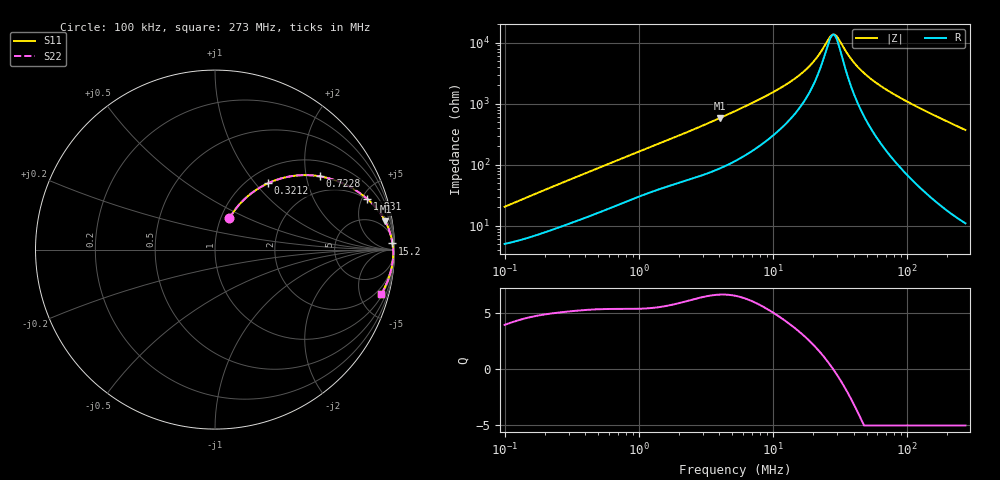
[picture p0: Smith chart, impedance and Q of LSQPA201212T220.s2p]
! LSQPA201212T220  S-PARAMETER MODEL  ( General Type )
! Model Generated by TAIYO YUDEN Corporation (http://www.ty-top.com)
! Version 2.0
! TAIYO YUDEN Control No. 100810NF17SB-FAC
! Copyright(c) 2007 TAIYO YUDEN CO.,LTD. All Rights Reserved.
! Product Description (link to TY-COMPAS)
! https://ds.yuden.co.jp/TYCOMPAS/or/detail?pn=LSQPA201212T220K&u=M
! Products Name : Inductors
! Characteristics :
!  Inductance : 22 uH , SRF(min) : 16 MHz , DC Resistance(max) : 4.81 Ohm
!  Rated Current : Saturation :170 mA , Temp Rise : 190 mA (40 degC)
!  Case Size : 2.0 x 1.25 / 0.079 x 0.049 [mm/inch] , Thickness : 1.25 / 0.049 [mm/inch]
!  (Conditions: Temperature = 25 degC , DC Bias Current/Voltage = 0A / 0V)
! External Node Assignments :
!  1  o---GGG---o  2
! GND o---------o GND
! Frequency Range : 0.1MHz  -  272.98108MHz  [ 402 STEP ]
# MHz S RI R 50
! Freq[MHz].  S11 Real  S11 Imag  S21 Real  S21 Imag  S12 Real  S12 Imag  S22 Real  S22 Imag
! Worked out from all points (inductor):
!   401 points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, 100 kHz to 273 MHz, reference 50 ohm
!   read as one part in series: L = 31.2 uH near 104 kHz
!   highest Q = 6.63 at 4.04 MHz (marker M1), where L = 22.8 uH
!   self-resonance near 28.07 MHz
!   S11 on the Smith chart (normalised r, x): 100 kHz: 1.10, +0.40; 321.2 kHz: 1.23, +1.17; 722.8 kHz: 1.45, +2.41; 1.831 MHz: 1.95, +5.48; 15.2 MHz: 16, +53; 273 MHz: 1.22, -7.41
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0.1  0.0807 0.1735  0.9193 -0.1735  0.9193 -0.1735  0.0807 0.1735
0.184629  0.1595 0.2765  0.8405 -0.2765  0.8405 -0.2765  0.1595 0.2765
0.32124  0.2956 0.3696  0.7044 -0.3696  0.7044 -0.3696  0.2956 0.3696
0.376316  0.3466 0.3899  0.6534 -0.3899  0.6534 -0.3899  0.3466 0.3899
0.722825  0.5858 0.408  0.4142 -0.408  0.4142 -0.408  0.5858 0.408
1.416134  0.7918 0.3253  0.2082 -0.3253  0.2082 -0.3253  0.7918 0.3253
1.831381  0.8478 0.2828  0.1522 -0.2828  0.1522 -0.2828  0.8478 0.2828
4.040099  0.9493 0.1566  0.0507 -0.1566  0.0507 -0.1566  0.9493 0.1566
5.329134  0.9654 0.1213  0.0346 -0.1213  0.0346 -0.1213  0.9654 0.1213
10.03569  0.9837 0.0617  0.0163 -0.0617  0.0163 -0.0617  0.9837 0.0617
15.20352  0.9889 0.0341  0.0111 -0.0341  0.0111 -0.0341  0.9889 0.0341
19.66158  0.991 0.0195  0.00903 -0.0195  0.00903 -0.0195  0.991 0.0195
22.13913  0.9917 0.013  0.00832 -0.013  0.00832 -0.013  0.9917 0.013
26.45291  0.9925 0.00346  0.0075 -0.00346  0.0075 -0.00346  0.9925 0.00346
28.63088  0.9928 -0.0008  0.00723 0.0008  0.00723 0.0008  0.9928 -0.0008
30.38126  0.9929 -0.00402  0.00707 0.00402  0.00707 0.00402  0.9929 -0.00402
37.0262  0.9932 -0.015  0.00679 0.015  0.00679 0.015  0.9932 -0.015
44.24071  0.9931 -0.0255  0.00688 0.0255  0.00688 0.0255  0.9931 -0.0255
54.99405  0.9925 -0.0396  0.00752 0.0396  0.00752 0.0396  0.9925 -0.0396
73.9896  0.9904 -0.0618  0.00961 0.0618  0.00961 0.0618  0.9904 -0.0618
133.9308  0.9783 -0.1241  0.0217 0.1241  0.0217 0.1241  0.9783 -0.1241
272.9811  0.9259 -0.2476  0.0741 0.2476  0.0741 0.2476  0.9259 -0.2476
